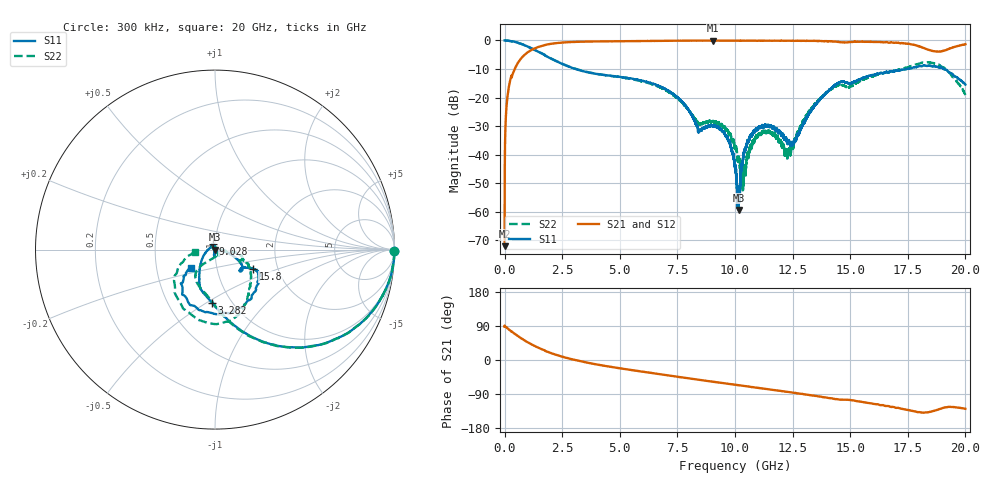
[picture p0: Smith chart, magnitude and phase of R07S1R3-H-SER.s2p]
!{R07S1R3}
!Johanson Technology Inc.
!www.johansontechnology.com
!Test Board Conditions:
!Substrate Type  RO4350B
!Substrate Thickness  10 mil
!Substrate Dk  3.66
!TL Type: GCPW
!TL Trace Width  21 mil
!TL Gap  20 mil
!Electrode orientation  Horizontal
!DUT TOPOLOGY	SERIES
!Mounting Pad LxW  16x21 mil
! Created Sat Feb  6 11:17:28 2021
# hz S ma R 50
! 2 Port Network Data from SP1.SP block
! freq  magS11  angS11  magS21  angS21  magS12  angS12  magS22  angS22
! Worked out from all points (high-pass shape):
!   20001 points, 300 kHz to 20 GHz, reference 50 ohm
!   highest |S21| = -0.05 dB at 9.058 GHz (marker M1); lowest = -72.1 dB at 300 kHz (marker M2)
!   |S21| within 3 dB of the highest: 1.232 GHz to 18.31 GHz (17.08 GHz wide, 175 % of centre); 19.25 GHz to end of sweep
!   lowest |S11| = -59.4 dB at 10.15 GHz (marker M3), VSWR 1.00, Z = 49.9 - j0.0245 ohm
!   |S11| at or under -10 dB: 3.086 GHz to 17.46 GHz (14.37 GHz wide, 140 % of centre); 19.05 GHz to end of sweep
!   |S22| runs from -52.5 to 0.0 dB; largest |S21 - S12| = 0.015
!   S11 on the Smith chart (normalised r, x): 300 kHz: open; 3.282 GHz: 0.81, -0.53; 9.028 GHz: 0.97, +0.06; 15.8 GHz: 1.50, -0.34; 20 GHz: 0.75, -0.16
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300000  1 -0.5  0.0002482 87.5  0.0003077 87.0  1 -0.6
1.343e8  0.9934 -7.1  0.1122 83.2  0.1121 83.2  0.9924 -7.1
5.063e8  0.9297 -23.5  0.3602 66.2  0.3601 66.1  0.9311 -23.4
1.8503e9  0.521 -67.8  0.8505 21.7  0.8507 21.8  0.5212 -68.1
3.2823e9  0.2984 -92.9  0.9498 -3.1  0.95 -3.1  0.3003 -91.6
3.3343e9  0.2943 -93.5  0.9508 -3.8  0.9503 -3.8  0.297 -92.3
6.6673e9  0.1616 -122.9  0.9841 -36.8  0.9837 -36.9  0.1558 -130.8
8.4593e9  0.02581 141.2  0.9931 -52.4  0.9918 -52.5  0.03399 -76.0
9.0283e9  0.03172 112.6  0.9939 -57.2  0.9938 -57.3  0.03839 -55.9
9.0583e9  0.03074 110.4  0.9948 -57.5  0.9938 -57.5  0.03756 -52.9
9.6953e9  0.01791 100.5  0.9922 -62.7  0.9907 -62.8  0.02632 -51.1
1.00003e10  0.006245 110.6  0.9934 -65.2  0.9931 -65.3  0.01224 -61.6
1.01533e10  0.001069 -166.7  0.9914 -66.5  0.9907 -66.5  0.008064 -80.8
1.03723e10  0.01055 -99.7  0.9915 -68.2  0.9912 -68.3  0.004137 -177.8
1.08503e10  0.02518 -96.1  0.992 -72.1  0.9915 -72.2  0.01787 138.1
1.15203e10  0.03158 -99.6  0.9894 -77.8  0.9893 -77.9  0.02408 125.7
1.23393e10  0.01785 -69.6  0.9885 -84.6  0.9888 -84.6  0.01221 52.2
1.33343e10  0.06127 -11.7  0.983 -93.3  0.9827 -93.4  0.06646 -7.4
1.58003e10  0.2394 -26.6  0.9472 -113.4  0.9447 -113.6  0.2257 -29.6
1.66673e10  0.2749 -29.2  0.915 -121.8  0.9202 -122.3  0.2803 -45.3
1.86273e10  0.3515 -98.1  0.6491 -134.3  0.6489 -134.5  0.399 -104.7
2e10  0.1688 -143.3  0.8605 -128.8  0.8582 -128.7  0.1106 -172.0
